(* Logix 5000 DataType export Banner_Direct_v4; software revision 33.00 *)

TYPE Banner_Direct_v4 :
STRUCT
   Master_Cycle_Time : INT;
   Min_Cycle_Time : INT;
   M_Sequence_Capability : INT;
   IO_Link_Version_ID : INT;
   Process_Data_Input_Length : INT;
   Process_Data_Output_Length : INT;
   Combined_Vendor_ID : DINT;   // IO-Link Vendor ID
   Vendor_ID1 : INT;
   Vendor_ID2 : INT;
   Combined_Device_ID : DINT;   // IO-Link Device ID
   Device_ID1 : INT;
   Device_ID2 : INT;
   Device_ID3 : INT;
END_STRUCT
END_TYPE
